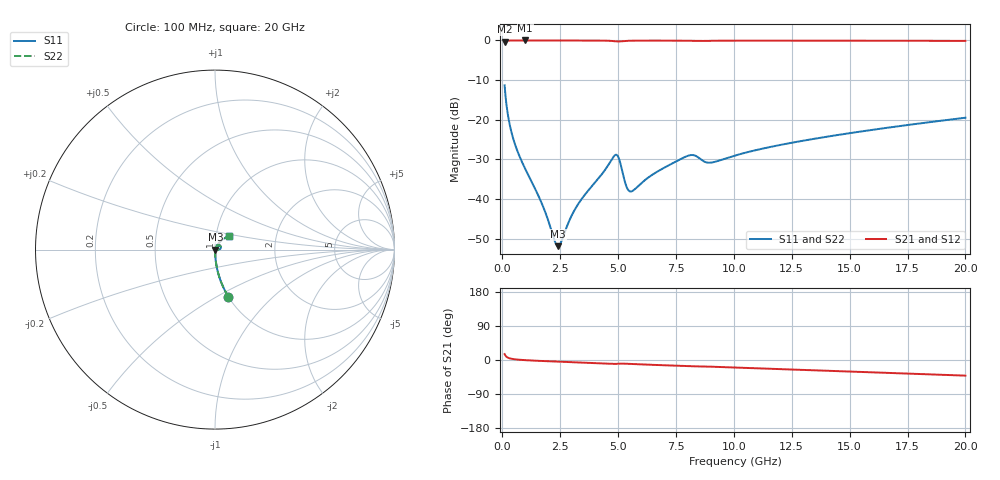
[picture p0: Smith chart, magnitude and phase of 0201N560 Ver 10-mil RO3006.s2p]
# GHz S MA R 50
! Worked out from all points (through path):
!   1601 points, 100 MHz to 20 GHz, reference 50 ohm
!   highest |S21| = -0.02 dB at 983.1 MHz (marker M1); lowest = -0.3 dB at 100 MHz (marker M2)
!   group delay of S21, straight-line fit = 5.93 ps
!   lowest |S11| = -51.9 dB at 2.413 GHz (marker M3), VSWR 1.01, Z = 50.3 - j0.0295 ohm
!   |S11| at or under -10 dB: start of sweep to end of sweep
!   |S22| runs from -51.9 to -11.3 dB; largest |S21 - S12| = 0
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0.1  0.2722 -74.2  0.9614 15.6  0.9614 15.6  0.2722 -74.2
0.274125  0.1016 -84.1  0.9938 5.3  0.9938 5.3  0.1016 -84.1
0.423375  0.06483 -86.1  0.9968 3.0  0.9968 3.0  0.06483 -86.1
0.64725  0.04075 -87.0  0.9978 1.2  0.9978 1.2  0.04075 -87.0
0.9830625  0.02429 -86.6  0.9981 -0.4  0.9981 -0.4  0.02429 -86.6
1.667125  0.009381 -79.6  0.9978 -2.5  0.9978 -2.5  0.009381 -79.6
2.264125  0.002968 -38.0  0.9975 -4.0  0.9975 -4.0  0.002968 -38.0
2.413375  0.002554 -6.6  0.9974 -4.3  0.9974 -4.3  0.002554 -6.6
2.550187  0.002925 21.0  0.9973 -4.7  0.9973 -4.7  0.002925 21.0
3.022813  0.006438 56.9  0.9969 -5.8  0.9969 -5.8  0.006438 56.9
3.420812  0.009975 63.9  0.9966 -6.7  0.9966 -6.7  0.009975 63.9
4.876  0.03597 36.2  0.9747 -10.3  0.9747 -10.3  0.03597 36.2
5.02525  0.03313 14.3  0.9695 -9.8  0.9695 -9.8  0.03313 14.3
5.348625  0.01475 8.8  0.9859 -9.9  0.9859 -9.9  0.01475 8.8
5.52275  0.01249 27.8  0.99 -10.4  0.99 -10.4  0.01249 27.8
6.741625  0.02261 62.1  0.9939 -13.3  0.9939 -13.3  0.02261 62.1
8.097312  0.03571 52.1  0.9861 -16.4  0.9861 -16.4  0.03571 52.1
8.943062  0.02874 48.8  0.9879 -17.5  0.9879 -17.5  0.02874 48.8
10.05  0.03539 59.0  0.9924 -20.0  0.9924 -20.0  0.03539 59.0
13.37081  0.05691 56.6  0.9918 -27.0  0.9918 -27.0  0.05691 56.6
16.69162  0.07976 51.0  0.9895 -34.1  0.9895 -34.1  0.07976 51.0
20  0.106 44.7  0.9863 -41.2  0.9863 -41.2  0.106 44.7
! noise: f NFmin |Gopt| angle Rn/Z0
0.1  0.000598  0.9283  0.2249  0.001853
2.301  0.004729  0.8049  4.143  0.00503
4.515  0.0122  0.8483  8.096  0.01704
6.729  0.01223  0.7829  12.03  0.01144
8.943  0.02012  0.8215  15.98  0.02317
11.14  0.01648  0.7414  19.78  0.01241
13.36  0.01817  0.7232  23.59  0.01249
15.57  0.02018  0.7129  27.37  0.01311
17.79  0.02225  0.7057  31.09  0.01381
20  0.02433  0.7004  34.77  0.01452
